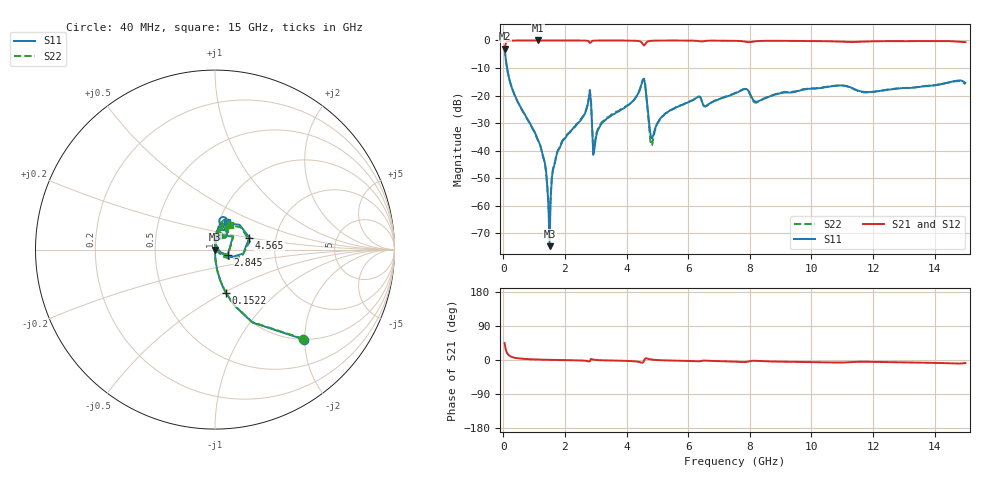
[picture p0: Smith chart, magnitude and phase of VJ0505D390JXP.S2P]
! VJ0505D390JXP
! MLCC placed on 25 mil thick microstrip substrate in series configuraton.
! DATE 06/29/2018  09:18
! CORRECTED  DATA
# GHz  S  MA  R  50.00
!  FREQ  S11M  S11A  S21M  S21A  S12M  S12A  S22M  S22A
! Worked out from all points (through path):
!   401 points, 40 MHz to 15 GHz, reference 50 ohm
!   highest |S21| = -0.01 dB at 1.125 GHz (marker M1); lowest = -3.0 dB at 40 MHz (marker M2)
!   group delay of S21, straight-line fit = 2.19 ps
!   lowest |S11| = -74.7 dB at 1.499 GHz (marker M3), VSWR 1.00, Z = 50 - j0.0125 ohm
!   |S11| at or under -10 dB: 119.2 MHz to end of sweep
!   |S22| runs from -67.2 to -3.1 dB; largest |S21 - S12| = 0.0024
!   S11 on the Smith chart (normalised r, x): 40 MHz: 0.99, -1.99; 152.2 MHz: 1.00, -0.52; 2.845 GHz: 1.15, -0.07; 4.565 GHz: 1.46, +0.20; 15 GHz: 1.09, +0.35
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0.04  0.7066 -45.2  0.7094 44.8  0.7097 44.8  0.7003 -45.3
0.1522  0.2507 -75.7  0.9667 14.5  0.9672 14.6  0.2487 -75.8
1.1246  0.01542 -89.9  0.9984 1.2  0.9986 1.3  0.0152 -92.2
1.3116  0.007189 -90.8  0.9981 0.8  0.9986 0.9  0.007066 -95.4
1.4986  0.000185 -42.4  0.9978 0.4  0.9984 0.5  0.0004357 171.1
1.6482  0.005288 88.2  0.9979 0.2  0.998 0.2  0.005566 93.3
1.7978  0.01054 87.7  0.9971 -0.1  0.9976 0.0  0.01082 90.3
2.5458  0.03833 86.4  0.9948 -1.3  0.9954 -1.3  0.0394 85.5
2.7702  0.08628 67.9  0.9665 -3.8  0.967 -3.8  0.08818 67.6
2.845  0.07695 -23.0  0.9275 2.9  0.9277 3.0  0.07845 -22.6
2.9946  0.01603 79.7  0.9942 0.1  0.9946 0.1  0.01715 76.5
3.219  0.03251 88.2  0.9959 -0.8  0.9963 -0.7  0.034 86.7
4.5654  0.2028 19.3  0.8069 -2.2  0.8076 -2.1  0.1988 13.2
4.7898  0.01752 10.5  0.9831 1.4  0.9836 1.5  0.01255 6.3
5.0516  0.03521 82.0  0.9933 -0.4  0.9938 -0.3  0.03431 84.7
6.2858  0.09214 79.1  0.9809 -3.4  0.9813 -3.4  0.09195 77.9
6.585  0.06466 78.1  0.9836 -1.8  0.9842 -1.7  0.0647 76.5
7.52  0.1093 83.1  0.984 -4.4  0.9848 -4.4  0.1112 80.2
8.2306  0.0771 68.6  0.9703 -2.3  0.9708 -2.3  0.07506 68.3
10.0258  0.1337 78.7  0.9697 -5.7  0.9713 -5.8  0.1351 73.6
12.5316  0.1281 76.2  0.9696 -5.7  0.9702 -5.7  0.129 73.6
15  0.1696 66.5  0.9306 -8.0  0.9313 -8.0  0.1602 58.5
